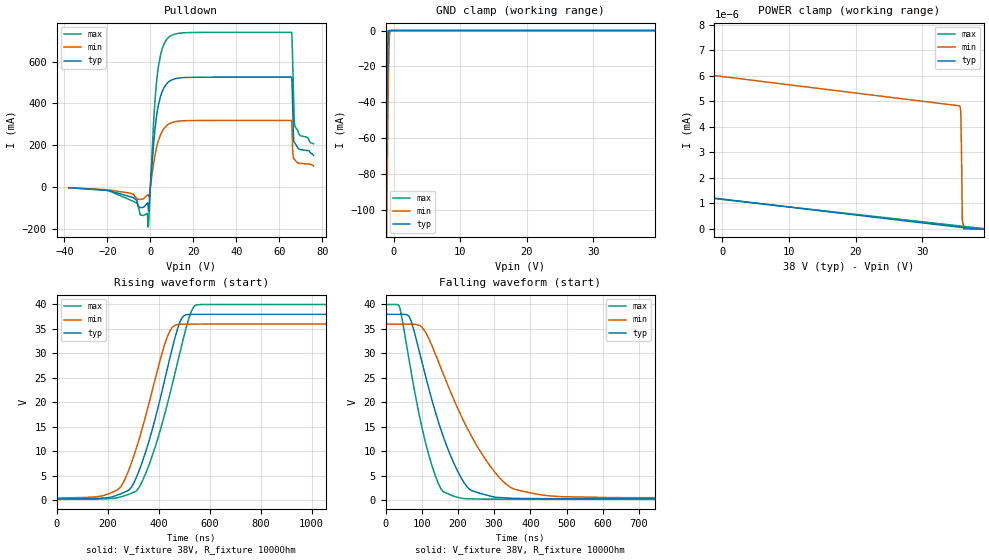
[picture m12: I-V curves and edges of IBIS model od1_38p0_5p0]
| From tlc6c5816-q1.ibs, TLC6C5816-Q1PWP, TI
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|   od1_38p0_5p0 Model
[Model]   od1_38p0_5p0
Model_type   Open_drain
Polarity   Inverting
Vmeas = 19
Vref = 38
Cref = 2pF
Rref = 1000
|   typ   min   max
C_comp   2.628pF   2.247pF   2.752pF
| Where Nom  PVT is Nominal Process, 38.0V, 27C
|   Fast PVT is Strong Process,  40.0V, -40C
|   Slow PVT is Weak Process,   36.0V, 150C
[Voltage Range]   38   36   40
|Junction Temperature
[Temperature Range]   27   150   -40
[Pullup Reference]   38   36   40
[Pulldown Reference]   0   -0   0
[Power Clamp Reference]   38   36   40
[GND Clamp Reference]   0   0   0
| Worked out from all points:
|   slope of the pulldown table from 0 to 5.7 V, typ, clamps not added: 12.4 ohm
|   GND clamp passes 1 mA (typ) near -0.73 V on its own axis
|   falling waveform, V_fixture 38V, R_fixture 1000Ohm: 20-80 % time 94.1ns typ, 140ns min, 66.6ns max; typ from 38 V to 0.262 V
|   rising waveform, V_fixture 38V, R_fixture 1000Ohm: 20-80 % time 115ns typ, 114ns min, 124ns max; typ from 0.262 V to 38 V
[Pulldown]
|   Voltage   I(typ)   I(min)   I(max)
-38V      -2.874mA   -2.999mA   -2.841mA
-7.904V   -50.9mA    -34.24mA   -68.15mA
-1.52V    -78.06mA   -39.42mA   -125.2mA
-950mV    -102.9mA   -36.14mA   -191.4mA
1.672V    225.2mA    122.1mA    337.7mA
3.724V    390.5mA    222.1mA    574mA
6.46V     477.3mA    281.4mA    686.3mA
12.84V    520.8mA    315mA      734.7mA
65.74V    525.7mA    317.2mA    739.9mA
66.65V    243.1mA    140.2mA    452.3mA
67.22V    210.9mA    130.8mA    293.1mA
76V       152.7mA    101.2mA    207.5mA
[GND Clamp]
|   Voltage   I(typ)   I(min)   I(max)
-38V      -18.95A    -18.51A    -19.22A
-1.292V   -161.2mA   -209.4mA   -136.1mA
-1.178V   -117.5mA   -166.8mA   -91.39mA
-1.064V   -75.38mA   -125.1mA   -48.96mA
-950mV    -36.53mA   -85.06mA   -13.12mA
-836mV    -7.654mA   -48.07mA   -310uA
-722mV    -266uA     -17.89mA   -2.372uA
-608mV    -5.048uA   -2.691mA   -37.32nA
-494mV    -96.2nA    -186.5uA   -1.113nA
-266mV    -44.51pA   -662nA     -4.297pA
76V       0A         0A         0A
[POWER Clamp]
|   Voltage   I(typ)   I(min)   I(max)
-38V      4.427A     3.422A     5.462A
-29.56V   655.6mA    11.74uA    1.527A
-28.77V   333.6mA    6.877nA    1.172A
-27.85V   4.302mA    6.854nA    781mA
-26.49V   1.98nA     6.818nA    220.5mA
-9.5V     1.468nA    6.276nA    1.433nA
35.53V    68.2pA     4.821nA    120.6pA
35.76V    61.3pA     4.592nA    114pA
35.87V    57.85pA    2.841nA    110.7pA
35.99V    54.41pA    348.9pA    107.5pA
36.21V    47.53pA    0A         100.9pA
76V       0A         0A         0A
[Ramp]
R_load = 1000
|   typ   min   max
dV/dt_r   22.643/1.14796e-07   21.326/1.14173e-07   23.8889/1.23433e-07
dV/dt_f   22.643/9.4016e-08   21.326/1.40246e-07   23.8889/6.65978e-08
[Falling Waveform]
V_fixture = 38V
V_fixture_min = 36V
V_fixture_max = 40V
R_fixture = 1000Ohm
C_fixture = 0F
|   Time   V(typ)   V(min)   V(max)
0s        38V        36V        40V
39.42ns   37.99V     35.98V     39.32V
66.81ns   37.31V     35.97V     27.91V
103.3ns   27.49V     35.13V     14.03V
138.8ns   17.77V     29.66V     4.759V
159.1ns   13.12V     25.91V     1.769V
208.2ns   4.661V     17.36V     424.2mV
326.4ns   500.4mV    3.725V     217.1mV
452ns     315.7mV    894.9mV    197.6mV
2.5us     261.7mV    456.7mV    185.2mV
[Rising Waveform]
V_fixture = 38V
V_fixture_min = 36V
V_fixture_max = 40V
R_fixture = 1000Ohm
C_fixture = 0F
|   Time   V(typ)   V(min)   V(max)
0s        261.7mV    456.7mV    185.2mV
243.1ns   1.144V     2.287V     569.2mV
290.9ns   2.463V     7.242V     1.372V
316.7ns   5.142V     11.26V     2.133V
368.1ns   13.13V     20.97V     8.017V
443.3ns   28.85V     34.49V     21.5V
491.7ns   37.26V     35.98V     31.87V
528.1ns   37.97V     36V        38.59V
548.7ns   38V        36V        39.92V
2.5us     38V        36V        40V
